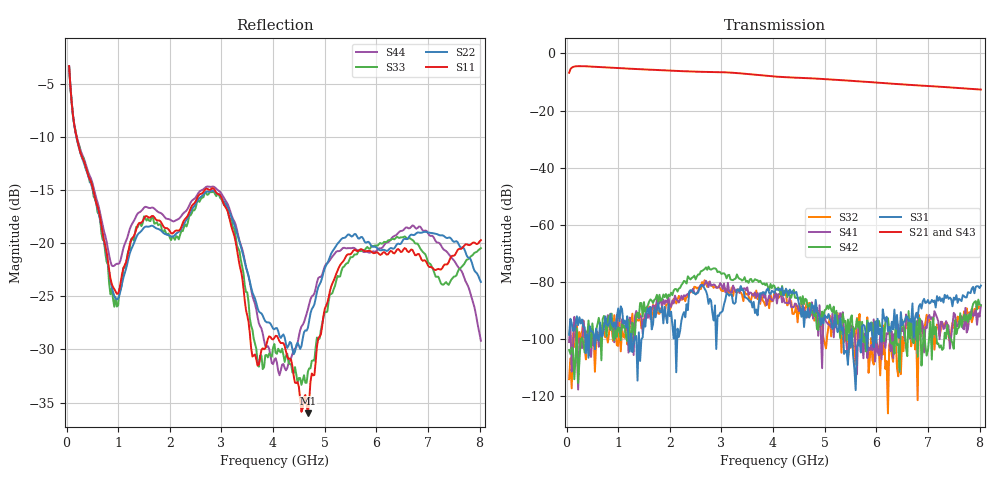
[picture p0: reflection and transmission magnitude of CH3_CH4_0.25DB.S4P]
!Agilent Technologies,E5071C,MY46316741,A.11.02
!Date: Thu May 28 15:05:14 2026
!Data & Calibration Information:
!1:CH3 INPUT 2:CH3 OUTPUT 3:CH4 INPUT 4:CH4 OUTPUT
!Freq	S11:SOLT4(ON)	S12:SOLT4(ON)	S13:SOLT4(ON)	S14:SOLT4(ON)
!	S21:SOLT4(ON)	S22:SOLT4(ON)	S23:SOLT4(ON)	S24:SOLT4(ON)
!	S31:SOLT4(ON)	S32:SOLT4(ON)	S33:SOLT4(ON)	S34:SOLT4(ON)
!	S41:SOLT4(ON)	S42:SOLT4(ON)	S43:SOLT4(ON)	S44:SOLT4(ON)
!PortZ  Port1:50+j0  Port2:50+j0  Port3:50+j0  Port4:50+j0
!Above PortZ is port z conversion or system Z0 setting when saving the data.
!When reading, reference impedance value at option line is always used.
# Hz S dB R 50
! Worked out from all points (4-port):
!   320 points, 50 MHz to 8.025 GHz, reference 50 ohm
!   strongest paths, dB at 50 MHz, 2.05 GHz, 4.05 GHz, 6.05 GHz, 8.025 GHz:
!     S21: -6.8, -6.0, -8.1, -10.2, -12.6
!     S43: -6.7, -6.1, -8.2, -10.4, -12.8
!     S31: -98.5, -94.9, -82.6, -98.3, -81.3
!     S42: -103.8, -84.6, -82.7, -93.6, -88.1
!     S41: -101.0, -86.4, -83.8, -105.7, -88.1
!     S32: -114.0, -87.2, -85.2, -103.9, -88.5
!   lowest |S11| = -36.0 dB at 4.675 GHz (marker M1), VSWR 1.03, Z = 48.7 - j0.896 ohm
!   |S11| at or under -10 dB: 194.3 MHz to end of sweep
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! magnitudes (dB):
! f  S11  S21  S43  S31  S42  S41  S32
! 50 MHz  -3.3  -6.8  -6.7  -98.5  -103.8  -101.0  -114.0
! 925 MHz  -24.3  -5.1  -5.1  -94.1  -100.3  -101.1  -91.6
! 2.85 GHz  -14.9  -6.5  -6.6  -93.4  -75.2  -80.8  -82.0
! 4.125 GHz  -29.2  -8.2  -8.3  -82.4  -82.9  -84.2  -85.2
! 4.675 GHz  -36.0  -8.7  -8.7  -89.2  -89.2  -91.8  -89.2
! 5.425 GHz  -21.1  -9.5  -9.5  -104.1  -100.4  -102.6  -98.9
! 8.025 GHz  -19.7  -12.6  -12.8  -81.3  -88.1  -88.1  -88.5
